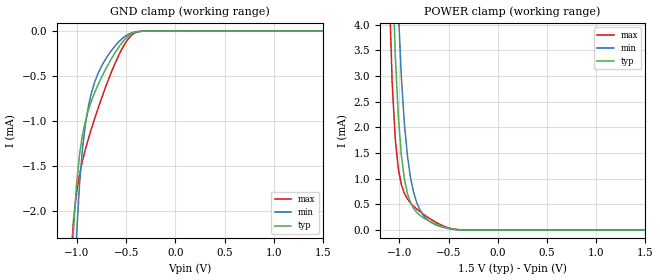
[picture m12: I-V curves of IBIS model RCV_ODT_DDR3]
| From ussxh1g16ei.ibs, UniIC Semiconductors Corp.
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|   Model RCV_ODT_DDR3
[Model] RCV_ODT_DDR3
Model_type Input
Vinl =  0.615V
Vinh =  0.885V
C_comp   0.902pF   0.902pF   0.902pF
[Model Spec]
Vinh   0.885V   0.847V   0.922V
Vinl   0.615V   0.577V   0.652V
[Temperature Range]   25.000   95.000   -40.000
[Voltage Range]   1.500V   1.425V   1.575V
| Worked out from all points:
|   GND clamp passes 1 mA (typ) near -0.91 V on its own axis
|   POWER clamp passes 1 mA (typ) near -0.95 V on its own axis
[GND_clamp]
|Voltage   I(typ)   I(min)   I(max)
-1.5V     -69.37mA   -68.94mA   -71.1mA
-1.066V   -3.056mA   -4.322mA   -2.621mA
-1.035V   -2.238mA   -3.131mA   -2.116mA
-1.004V   -1.714mA   -2.288mA   -1.806mA
-973mV    -1.376mA   -1.704mA   -1.598mA
-942mV    -1.149mA   -1.3mA     -1.44mA
-911mV    -989uA     -1.019mA   -1.307mA
-849mV    -766.8uA   -675.4uA   -1.076mA
-725mV    -460.8uA   -342.9uA   -673.5uA
-508mV    -86.33uA   -55.84uA   -133.3uA
-322mV    -1.052uA   -1.065uA   -1.064uA
1.5V      0A         0A         0A
[POWER_clamp]
|Voltage   I(typ)   I(min)   I(max)
-1.5V     89.87mA    92.1mA     88.82mA
-1.104V   7.876mA    11.84mA    4.749mA
-1.073V   5.259mA    8.664mA    2.865mA
-1.042V   3.423mA    6.175mA    1.777mA
-1.011V   2.217mA    4.314mA    1.194mA
-980mV    1.46mA     2.983mA    884.6uA
-949mV    995.9uA    2.065mA    712.2uA
-918mV    711.2uA    1.443mA    604.7uA
-856mV    421.6uA    739uA      466.2uA
-763mV    246.6uA    302.1uA    317.1uA
-391mV    4.434uA    4.343uA    4.369uA
1.5V      0A         0A         0A
